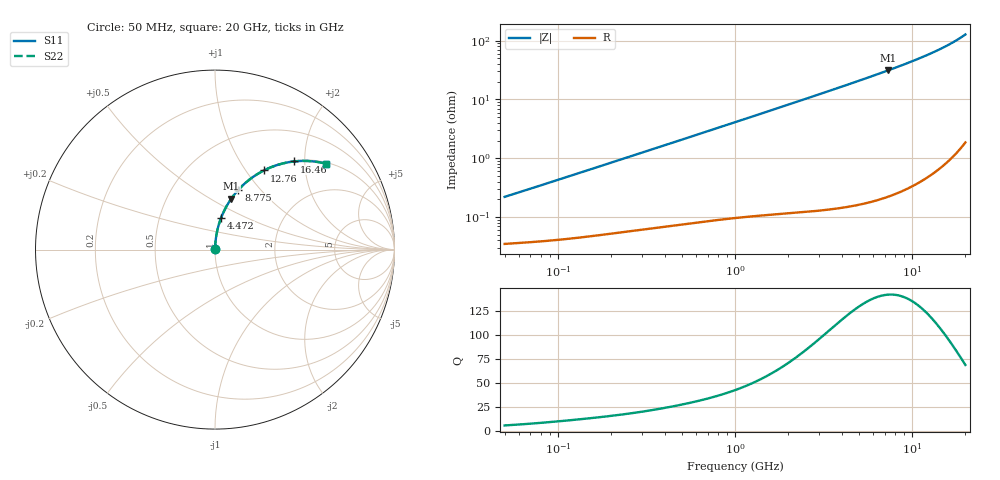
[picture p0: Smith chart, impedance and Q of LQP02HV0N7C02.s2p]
!Murata Part Number: LQP02HV0N7C02
!These Parameters are Measured in Series Mode Connection
!  o--[Z]--o
!Port1  Port2
!  o-------o
!Freq. Start=50[MHz] Stop=20[GHz], 401[Steps]
# Hz S RI R 50
!Freq.(Hz) S11(Real) S11(Imag) S21(Real) S21(Imag) S12(Real) S12(Imag) S22(Real) S22(Imag)
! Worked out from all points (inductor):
!   401 points, 50 MHz to 20 GHz, reference 50 ohm
!   read as one part in series: L = 686 pH near 51.52 MHz
!   highest Q = 141 at 7.331 GHz (marker M1), where L = 680 pH
!   S11 on the Smith chart (normalised r, x): 50 MHz: 1.00, +0.00; 4.472 GHz: 1.00, +0.37; 8.775 GHz: 1.01, +0.77; 12.76 GHz: 1.01, +1.22; 16.46 GHz: 1.02, +1.78; 20 GHz: 1.04, +2.56
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5e7  0.000352 0.00217  0.9996 -0.00217  0.9996 -0.00217  0.000352 0.00217
5.152053e7  0.000355 0.00223  0.9996 -0.00223  0.9996 -0.00223  0.000355 0.00223
6.07487e7  0.000368 0.00262  0.9996 -0.00262  0.9996 -0.00262  0.000368 0.00262
1.364002e8  0.000484 0.00577  0.9995 -0.00577  0.9995 -0.00577  0.000484 0.00577
3.721004e8  0.0009 0.0154  0.9991 -0.0154  0.9991 -0.0154  0.0009 0.0154
1e9  0.00263 0.0408  0.9974 -0.0408  0.9974 -0.0408  0.00263 0.0408
1.714689e9  0.00599 0.0696  0.994 -0.0696  0.994 -0.0696  0.00599 0.0696
2.728004e9  0.0135 0.1101  0.9865 -0.1101  0.9865 -0.1101  0.0135 0.1101
3.519108e9  0.0218 0.1414  0.9782 -0.1414  0.9782 -0.1414  0.0218 0.1414
4.472136e9  0.0345 0.1786  0.9655 -0.1786  0.9655 -0.1786  0.0345 0.1786
5.856089e9  0.0585 0.231  0.9415 -0.231  0.9415 -0.231  0.0585 0.231
7.331367e9  0.0911 0.2842  0.9089 -0.2842  0.9089 -0.2842  0.0911 0.2842
7.442007e9  0.0938 0.2881  0.9062 -0.2881  0.9062 -0.2881  0.0938 0.2881
8.774992e9  0.13 0.3328  0.87 -0.3328  0.87 -0.3328  0.13 0.3328
1.066139e10  0.1913 0.3895  0.8087 -0.3895  0.8087 -0.3895  0.1913 0.3895
1.166392e10  0.2283 0.4158  0.7717 -0.4158  0.7717 -0.4158  0.2283 0.4158
1.276073e10  0.2723 0.4409  0.7277 -0.4409  0.7277 -0.4409  0.2723 0.4409
1.460232e10  0.3531 0.4732  0.6469 -0.4732  0.6469 -0.4732  0.3531 0.4732
1.646126e10  0.4418 0.4912  0.5582 -0.4912  0.5582 -0.4912  0.4418 0.4912
1.800918e10  0.5189 0.4936  0.4811 -0.4936  0.4811 -0.4936  0.5189 0.4936
1.940974e10  0.5895 0.4851  0.4105 -0.4851  0.4105 -0.4851  0.5895 0.4851
2e10  0.619 0.4784  0.381 -0.4784  0.381 -0.4784  0.619 0.4784
